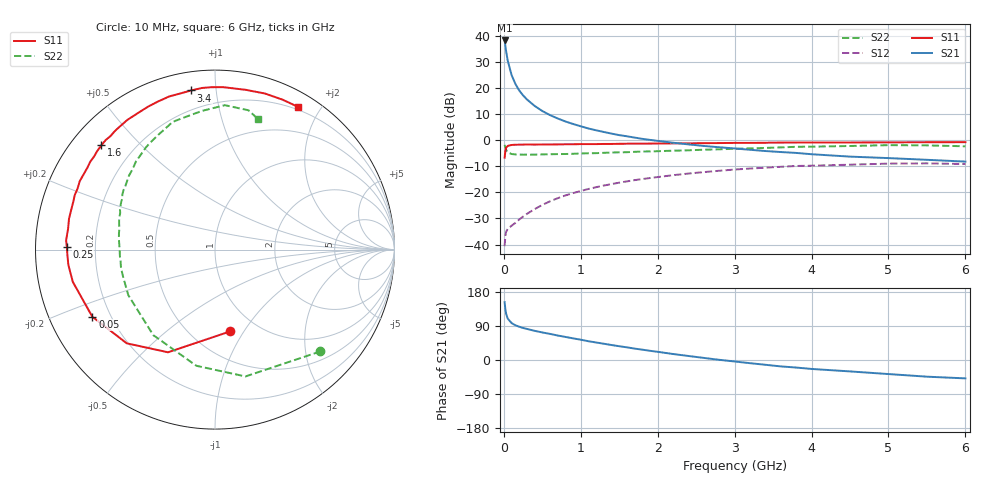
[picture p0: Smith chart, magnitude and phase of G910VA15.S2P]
! SIEMENS Small Signal Semiconductors
! BFG235
! Si NPN RF Bipolar Junction Transistor in SOT223
! VCE = 10 V  IC = 150 mA
! Common Emitter S-Parameters:  July  1994
# GHz  S  MA  R  50
!  f  S11  S21  S12  S22
! GHz  MAG  ANG  MAG  ANG  MAG  ANG  MAG  ANG
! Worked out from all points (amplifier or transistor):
!   40 points, 10 MHz to 6 GHz, reference 50 ohm
!   highest |S21| = 38.3 dB at 10 MHz (marker M1)
!   |S21| within 3 dB of that: start of sweep to 24.45 MHz
!   unconditionally stable (mu >= 1): 471.3 MHz to 1.49 GHz
!   at 200 MHz: K = 0.79, MSG = 24.8 dB, |S12| = -30.4 dB
!   at 1.5 GHz: K = 1.00, MSG = 9.1 dB, |S12| = -16.3 dB
!   at 6 GHz: K = 0.89, MSG = 0.5 dB, |S12| = -9.1 dB
!   S11 on the Smith chart (normalised r, x): 10 MHz: 0.75, -0.87; 50 MHz: 0.13, -0.25; 250 MHz: 0.10, +0.01; 1.6 GHz: 0.09, +0.39; 3.4 GHz: 0.09, +0.86; 6 GHz: 0.17, +1.73
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0.01  0.4637 -79.6  82.22 152.6  0.0093 62.7  0.8167 -44.0
0.02  0.6292 -114.6  64.78 133.7  0.0147 48.8  0.7268 -76.5
0.03  0.7173 -133.3  50.93 122.0  0.0176 41.6  0.6555 -99.1
0.05  0.7791 -151.3  33.98 109.4  0.0199 33.5  0.5877 -125.8
0.1  0.8123 -167.2  17.94 97.5  0.0229 36.2  0.5457 -152.2
0.15  0.8215 -174.1  12.07 91.6  0.026 42.6  0.5341 -163.1
0.2  0.8228 -177.7  9.028 87.8  0.0302 47.3  0.5336 -168.9
0.25  0.8256 178.9  7.266 84.5  0.0343 50.9  0.5302 -172.9
0.3  0.8311 176.5  6.07 82.0  0.0387 54.5  0.5311 -176.1
0.4  0.8267 171.9  4.563 77.0  0.0478 57.4  0.5312 179.5
0.5  0.8312 168.2  3.644 72.7  0.0575 59.3  0.5353 176.1
0.6  0.8312 165.1  3.042 68.9  0.0675 59.8  0.5394 173.0
0.7  0.8331 161.5  2.62 64.6  0.0774 59.8  0.543 170.2
0.9  0.8379 156.0  2.053 57.1  0.0969 58.0  0.551 165.7
1.1  0.8437 149.7  1.682 49.5  0.1163 55.5  0.5628 161.0
1.6  0.8595 137.4  1.193 33.4  0.1628 47.5  0.5904 150.9
2.2  0.8722 124.0  0.897 15.8  0.2139 36.8  0.6321 139.3
3.2  0.891 102.7  0.657 -8.4  0.2868 17.5  0.6987 120.5
3.4  0.8967 98.5  0.622 -12.6  0.2982 13.5  0.7136 116.2
4.5  0.9066 79.0  0.486 -30.1  0.3401 -7.4  0.7763 95.3
5.5  0.9163 65.7  0.422 -44.0  0.3604 -25.8  0.7983 76.5
6  0.9199 59.8  0.39 -48.5  0.3503 -32.6  0.7662 71.8
